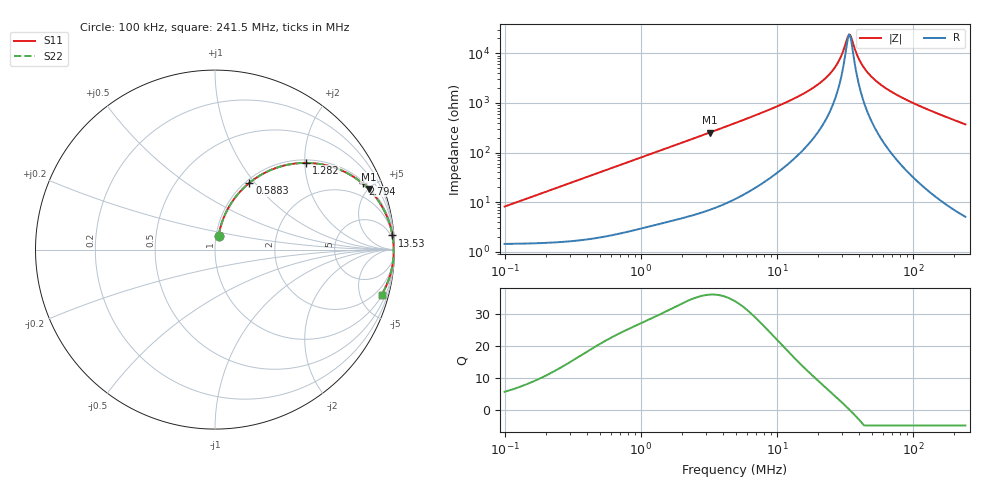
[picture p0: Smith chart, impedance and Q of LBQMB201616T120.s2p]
! LBQMB201616T120  S-PARAMETER MODEL  ( General Type )
! Model Generated by TAIYO YUDEN Corporation (http://www.ty-top.com)
! Version 1.0
! TAIYO YUDEN Control No. 191025NI43SB-FBB
! Copyright(c) 2019 TAIYO YUDEN CO.,LTD. All Rights Reserved.
! Product Description (link to TY-COMPAS)
! https://ds.yuden.co.jp/TYCOMPAS/or/detail?pn=LBQMB201616T120J&u=M
! Products Name : Inductors
! Characteristics :
!  Inductance : 12 uH , SRF(min) : 23 MHz , DC Resistance(max) : 1.82 Ohm , Rated Current : 200 mA
!  Case Size : 2.0 x 1.6 / 0.079 x 0.063 [mm/inch] , Thickness : 1.6 / 0.063 [mm/inch]
!  (Conditions: Temperature = 25 degC , DC Bias Current/Voltage = 0A / 0V)
! External Node Assignments :
!  1  o---GGG---o  2
! GND o---------o GND
! Frequency Range : 0.1MHz  -  241.513628MHz  [ 402 STEP ]
# MHz S RI R 50
! Freq[MHz].  S11 Real  S11 Imag  S21 Real  S21 Imag  S12 Real  S12 Imag  S22 Real  S22 Imag
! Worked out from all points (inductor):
!   401 points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, 100 kHz to 241.5 MHz, reference 50 ohm
!   read as one part in series: L = 12.8 uH near 104 kHz
!   highest Q = 36.2 at 3.202 MHz (marker M1), where L = 12.5 uH
!   self-resonance near 33.79 MHz
!   S11 on the Smith chart (normalised r, x): 100 kHz: 1.03, +0.16; 588.3 kHz: 1.04, +0.94; 1.282 MHz: 1.07, +2.03; 2.794 MHz: 1.12, +4.40; 13.53 MHz: 3, +25; 241.5 MHz: 1.10, -7.40
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0.1  0.0203 0.0776  0.9797 -0.0776  0.9797 -0.0776  0.0203 0.0776
0.368674  0.0933 0.2633  0.9067 -0.2633  0.9067 -0.2633  0.0933 0.2633
0.588328  0.1917 0.3719  0.8083 -0.3719  0.8083 -0.3719  0.1917 0.3719
1.282075  0.5069 0.4832  0.4931 -0.4832  0.4931 -0.4832  0.5069 0.4832
1.359207  0.5348 0.4823  0.4652 -0.4823  0.4652 -0.4823  0.5348 0.4823
2.793879  0.8221 0.3687  0.1779 -0.3687  0.1779 -0.3687  0.8221 0.3687
3.201909  0.8577 0.3358  0.1423 -0.3358  0.1423 -0.3358  0.8577 0.3358
4.914404  0.9327 0.2364  0.0673 -0.2364  0.0673 -0.2364  0.9327 0.2364
13.52861  0.9888 0.0786  0.0112 -0.0786  0.0112 -0.0786  0.9888 0.0786
18.11814  0.9928 0.0502  0.00723 -0.0502  0.00723 -0.0502  0.9928 0.0502
22.44628  0.9945 0.032  0.00554 -0.032  0.00554 -0.032  0.9945 0.032
26.2303  0.9952 0.0197  0.00476 -0.0197  0.00476 -0.0197  0.9952 0.0197
28.91279  0.9956 0.0122  0.00443 -0.0122  0.00443 -0.0122  0.9956 0.0122
32.49632  0.9958 0.00331  0.00418 -0.00331  0.00418 -0.00331  0.9958 0.00331
33.78694  0.9959 0.000366  0.00413 -0.000366  0.00413 -0.000366  0.9959 0.000366
35.12882  0.9959 -0.00258  0.0041 0.00258  0.0041 0.00258  0.9959 -0.00258
39.48278  0.9959 -0.0115  0.0041 0.0115  0.0041 0.0115  0.9959 -0.0115
44.37638  0.9957 -0.0206  0.00427 0.0206  0.00427 0.0206  0.9957 -0.0206
52.87715  0.9951 -0.0348  0.00488 0.0348  0.00488 0.0348  0.9951 -0.0348
66.79689  0.9935 -0.0555  0.00654 0.0555  0.00654 0.0555  0.9935 -0.0555
113.0069  0.9835 -0.1147  0.0165 0.1147  0.0165 0.1147  0.9835 -0.1147
241.5136  0.9289 -0.2502  0.0711 0.2502  0.0711 0.2502  0.9289 -0.2502
